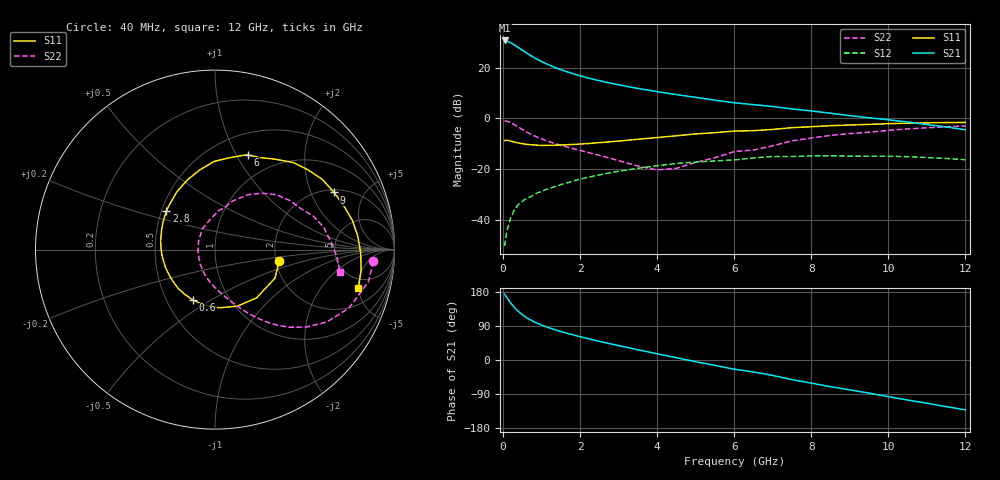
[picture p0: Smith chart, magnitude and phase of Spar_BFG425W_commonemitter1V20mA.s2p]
! Filename: 120bf425.001
! BFG425W Field C1
! V1=8.742E-001V,V2=1.000E+000V, I1=3.055E-004A, I2=2.001E-002A
# GHz  S  MA  R 50
!  S11  S21  S12  S22
!Freq(GHz)  Mag  Ang  Mag  Ang  Mag  Ang  Mag  Ang
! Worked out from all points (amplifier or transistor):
!   44 points, 40 MHz to 12 GHz, reference 50 ohm
!   highest |S21| = 30.7 dB at 40 MHz (marker M1)
!   |S21| within 3 dB of that: start of sweep to 416.6 MHz
!   unconditionally stable (mu >= 1): 1.182 GHz to end of sweep
!   at 700 MHz: K = 0.80, MSG = 28.0 dB, |S12| = -31.1 dB
!   at 2.4 GHz: K = 1.17, MAG = 16.4 dB, |S12| = -22.6 dB
!   at 12 GHz: K = 1.36, MAG = 2.3 dB, |S12| = -16.4 dB
!   S11 on the Smith chart (normalised r, x): 40 MHz: 2.09, -0.30; 600 MHz: 0.68, -0.42; 2.8 GHz: 0.53, +0.26; 6 GHz: 0.72, +1.11; 9 GHz: 2.13, +2.97; 12 GHz: 3.69, -4.97
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0.04  0.363 -9.8  34.24 173.6  0.003 77.3  0.885 -4.2
0.1  0.37 -25.4  33.3 164.4  0.006 81.2  0.873 -11.9
0.2  0.355 -49.3  30.68 149.9  0.011 73.3  0.815 -23.5
0.3  0.339 -68.5  27.79 138.1  0.016 68.4  0.742 -32.9
0.4  0.325 -86.0  24.72 128.0  0.02 64.2  0.667 -40.3
0.5  0.315 -101.3  21.95 119.4  0.023 61.3  0.6 -46.1
0.6  0.307 -113.6  19.55 112.4  0.026 59.7  0.543 -50.8
0.7  0.301 -123.9  17.52 106.5  0.028 58.1  0.494 -54.6
0.8  0.298 -133.1  15.81 101.2  0.031 57.3  0.454 -57.8
0.9  0.294 -141.0  14.38 96.5  0.034 56.4  0.42 -60.6
1.1  0.292 -154.2  12.09 88.4  0.039 54.8  0.367 -65.5
1.5  0.297 -174.4  9.098 75.2  0.049 51.8  0.293 -74.1
2.2  0.317 159.6  6.26 56.6  0.068 44.7  0.212 -89.9
2.8  0.345 141.7  4.898 42.5  0.085 37.1  0.161 -107.2
3.5  0.385 123.7  3.873 27.0  0.103 27.1  0.114 -137.6
4.5  0.451 101.2  2.934 6.0  0.128 11.5  0.103 153.0
6  0.559 71.1  2.024 -24.4  0.151 -13.3  0.22 84.3
6.5  0.569 64.3  1.857 -31.6  0.165 -17.4  0.237 77.8
8.5  0.714 33.3  1.258 -70.5  0.182 -53.4  0.459 41.8
9  0.736 25.7  1.126 -79.0  0.179 -61.3  0.5 32.9
10.5  0.799 5.5  0.843 -105.7  0.175 -86.8  0.617 11.8
12  0.827 -14.9  0.593 -131.7  0.152 -114.6  0.707 -10.2
